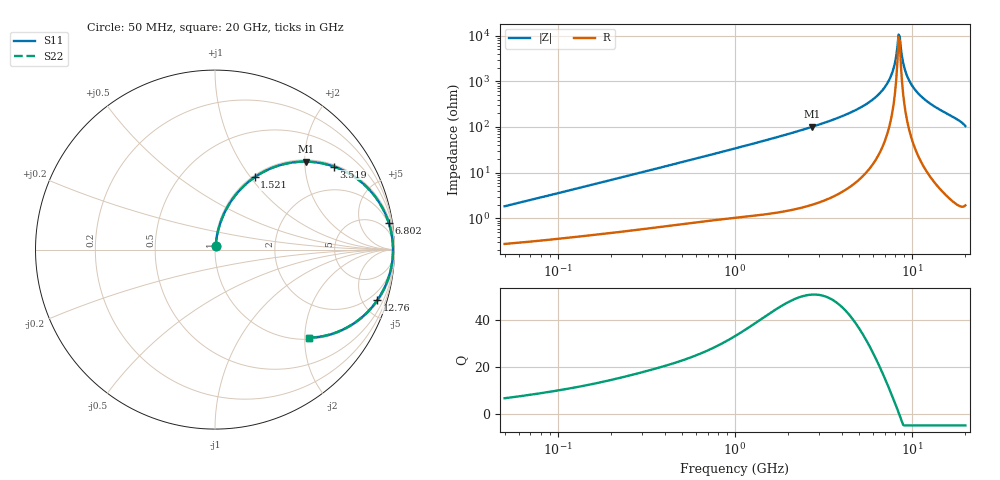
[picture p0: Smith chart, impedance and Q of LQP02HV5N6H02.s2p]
!Murata Part Number: LQP02HV5N6H02
!These Parameters are Measured in Series Mode Connection
!  o--[Z]--o
!Port1  Port2
!  o-------o
!Freq. Start=50[MHz] Stop=20[GHz], 401[Steps]
# Hz S RI R 50
!Freq.(Hz) S11(Real) S11(Imag) S21(Real) S21(Imag) S12(Real) S12(Imag) S22(Real) S22(Imag)
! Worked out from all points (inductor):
!   401 points, 50 MHz to 20 GHz, reference 50 ohm
!   read as one part in series: L = 5.74 nH near 51.52 MHz
!   highest Q = 50.8 at 2.728 GHz (marker M1), where L = 5.9 nH
!   self-resonance near 8.389 GHz
!   S11 on the Smith chart (normalised r, x): 50 MHz: 1.01, +0.04; 1.521 GHz: 1.02, +1.05; 3.519 GHz: 1.06, +2.82; 6.802 GHz: 2, +13; 12.76 GHz: 1.16, -6.36; 20 GHz: 1.04, -2.10
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5e7  0.00309 0.0182  0.9969 -0.0182  0.9969 -0.0182  0.00309 0.0182
1.364002e8  0.00631 0.0473  0.9937 -0.0473  0.9937 -0.0473  0.00631 0.0473
3.721004e8  0.022 0.1235  0.978 -0.1235  0.978 -0.1235  0.022 0.1235
1e9  0.1104 0.2986  0.8896 -0.2986  0.8896 -0.2986  0.1104 0.2986
1.521052e9  0.2206 0.4029  0.7794 -0.4029  0.7794 -0.4029  0.2206 0.4029
2.728004e9  0.5052 0.4902  0.4948 -0.4902  0.4948 -0.4902  0.5052 0.4902
3.519108e9  0.6626 0.4627  0.3374 -0.4627  0.3374 -0.4627  0.6626 0.4627
5.273168e9  0.8838 0.3061  0.1162 -0.3061  0.1162 -0.3061  0.8838 0.3061
6.125241e9  0.94 0.2182  0.06 -0.2182  0.06 -0.2182  0.94 0.2182
6.802353e9  0.9678 0.1501  0.0322 -0.1501  0.0322 -0.1501  0.9678 0.1501
7.442007e9  0.9834 0.0888  0.0166 -0.0888  0.0166 -0.0888  0.9834 0.0888
7.901521e9  0.9894 0.0468  0.0106 -0.0468  0.0106 -0.0468  0.9894 0.0468
8.264682e9  0.9915 0.015  0.00851 -0.015  0.00851 -0.015  0.9915 0.015
8.389408e9  0.9917 0.00439  0.00827 -0.00439  0.00827 -0.00439  0.9917 0.00439
8.516016e9  0.9917 -0.00626  0.00825 0.00626  0.00825 0.00626  0.9917 -0.00626
8.644534e9  0.9915 -0.0169  0.00846 0.0169  0.00846 0.0169  0.9915 -0.0169
9.041845e9  0.9895 -0.0489  0.0105 0.0489  0.0105 0.0489  0.9895 -0.0489
9.745021e9  0.9815 -0.1019  0.0185 0.1019  0.0185 0.1019  0.9815 -0.1019
1.082228e10  0.9604 -0.1747  0.0396 0.1747  0.0396 0.1747  0.9604 -0.1747
1.276073e10  0.9043 -0.2822  0.0957 0.2822  0.0957 0.2822  0.9043 -0.2822
1.670968e10  0.7463 -0.428  0.2537 0.428  0.2537 0.428  0.7463 -0.428
2e10  0.5233 -0.4903  0.4767 0.4903  0.4767 0.4903  0.5233 -0.4903
